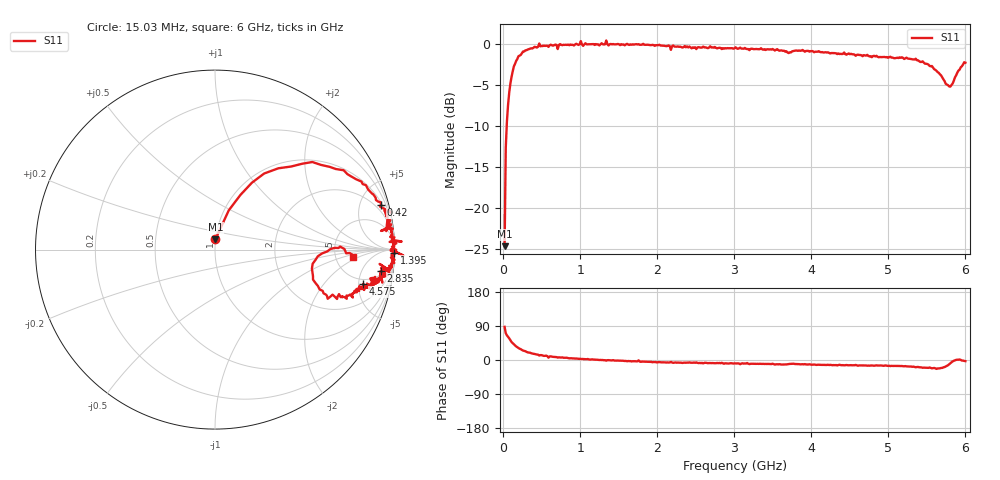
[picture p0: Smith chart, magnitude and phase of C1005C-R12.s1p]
!	Network	Analyzer	HP8753E.07.74:	Oct	30	2002	Serial	No.	JP38451487
!	Hewlett-Packard
!	28	Aug	2009	9:23:40
!	Frequency	S11
#	HZ	S	RI	R	50
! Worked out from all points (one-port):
!   400 points, 15.03 MHz to 6 GHz, reference 50 ohm
!   lowest |S11| = -24.7 dB at 15.03 MHz (marker M1), VSWR 1.12, Z = 49.9 + j5.84 ohm
!   |S11| at or under -10 dB: start of sweep to 42.53 MHz
!   S11 on the Smith chart (normalised r, x): 15.03 MHz: 1.00, +0.12; 420 MHz: 1.26, +7.37; 1.395 GHz: open; 2.835 GHz: 7, -12; 4.575 GHz: 4.22, -5.69; 6 GHz: 7.38, -1.42
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1.502992e7  0.00258 0.0583
3.002985e7  0.0769 0.219
6.00297e7  0.206 0.373
9.002955e7  0.353 0.453
1.95029e8  0.717 0.442
4.200279e8  0.924 0.248
4.650277e8  0.986 0.206
5.550272e8  0.956 0.196
5.850271e8  0.954 0.103
6.150269e8  0.976 0.164
7.050265e8  0.925 0.104
7.650262e8  0.976 0.119
1.005025e9  1.04 0.045
1.035025e9  0.973 0.0429
1.335023e9  1.05 -0.0333
1.395023e9  1 -0.0179
1.515022e9  0.983 -0.0312
2.265019e9  0.959 -0.115
2.835016e9  0.923 -0.119
3.015015e9  0.942 -0.152
3.765011e9  0.892 -0.152
4.515007e9  0.847 -0.204
4.575007e9  0.825 -0.191
5.265004e9  0.777 -0.24
5.625002e9  0.628 -0.274
5.790001e9  0.54 -0.106
5.895001e9  0.668 0.00977
6e9  0.768 -0.0393
